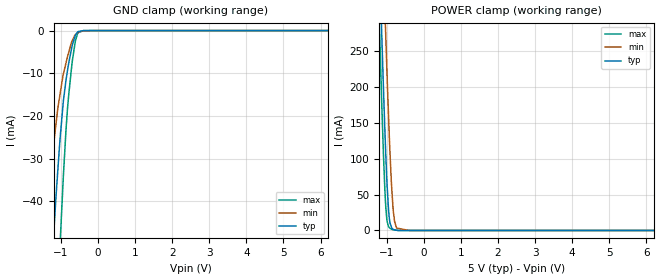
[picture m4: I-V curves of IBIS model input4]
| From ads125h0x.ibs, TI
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|   input4 Model
[Model]   input4
Model_type   Input
Vinl = 1.5
Vinh = 3.5
|   typ   min   max
C_comp   4.6952pF   3.83388pF   5.00796pF
|  Where Nom  PVT is Nominal Process,   5V,  27C
|   Fast PVT is Strong Process,   5.25V, -40C
|   Slow PVT is Weak Process,   2.7V, 135C
[Model spec]
|subparameter
Vinl   1.500   0.810   1.575
Vinh   3.500   1.890   3.675
[Voltage Range]   5   2.7   5.25
|Junction Temperature
[Temperature Range]   27   135   -40
[Power Clamp Reference]   5   2.7   5.25
[GND Clamp Reference]   0   0   0
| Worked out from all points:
|   GND clamp passes 1 mA (typ) near -0.61 V on its own axis
|   POWER clamp passes 1 mA (typ) near -0.79 V on its own axis
[GND Clamp]
|   Voltage   I(typ)   I(min)   I(max)
-5V       -779mA     -548.7mA   -950.6mA
-1.444V   -86.21mA   -48.51mA   -139.1mA
-1.25V    -55.46mA   -30.66mA   -96.43mA
-1.136V   -39.27mA   -22.07mA   -72.39mA
-1.022V   -25.14mA   -14.78mA   -49.76mA
-933.8mV  -16.44mA   -10.16mA   -33.97mA
-861.8mV  -11.49mA   -7.528mA   -22.97mA
-791.5mV  -7.679mA   -5.134mA   -15.13mA
-690.4mV  -3.28mA    -2.279mA   -6.94mA
-611.6mV  -1.099mA   -996.9uA   -2.485mA
-536.5mV  -236.8uA   -422.3uA   -497uA
10V       0A         0A         0A
[POWER Clamp]
|   Voltage   I(typ)   I(min)   I(max)
-5V       7.829A     7.978A     7.753A
-1.25V    473.6mA    653.3mA    374.5mA
-1.143V   287.8mA    464.7mA    190.9mA
-1.09V    198.8mA    373.8mA    106.6mA
-1.035V   118.1mA    284.7mA    40.75mA
-1.001V   74.07mA    230.7mA    16.66mA
-930.2mV  16.67mA    129.8mA    3.764mA
-876.6mV  5.132mA    67.8mA     2.053mA
-821.3mV  1.257mA    26mA       857.2uA
-735.3mV  423.1uA    3.33mA     277uA
-392.9mV  1.126uA    152.5nA    352.4nA
10V       0A         0A         0A
